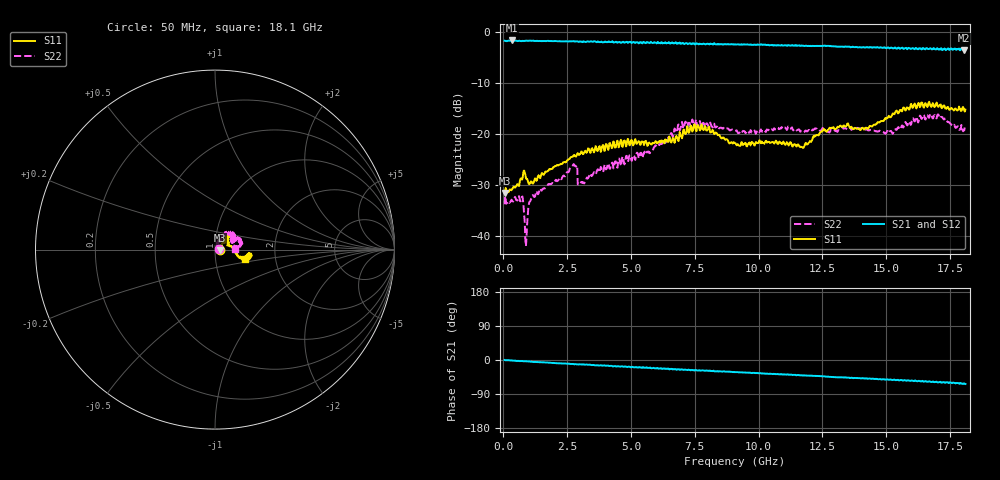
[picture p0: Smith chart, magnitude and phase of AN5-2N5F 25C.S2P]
! Network Analyzer HP8720D.06.14 Serial No. US36140669
! 12 Jan 2005  10:38:57
! Frequency  S11  S21  S12  S22
# HZ  S  DB R 50
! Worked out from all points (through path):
!   801 points, 50 MHz to 18.1 GHz, reference 50 ohm
!   highest |S21| = -1.60 dB at 343.3 MHz (marker M1); lowest = -3.5 dB at 18.03 GHz (marker M2)
!   group delay of S21, straight-line fit = 9.32 ps
!   lowest |S11| = -31.6 dB at 50 MHz (marker M3), VSWR 1.05, Z = 52.7 - j0.304 ohm
!   |S11| at or under -10 dB: start of sweep to end of sweep
!   |S22| runs from -42.0 to -16.0 dB; largest |S21 - S12| = 0.027
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5e7  -31.58 -6.3  -1.66 0.2  -1.68 -0.3  -33.79 4.1
3.433125e8  -30.75 12.3  -1.60 -1.5  -1.64 -1.7  -33.07 5.1
6.8175e8  -28.71 21.9  -1.72 -2.8  -1.70 -3.2  -33.19 10.7
8.848125e8  -28.68 10.7  -1.65 -3.3  -1.66 -3.7  -42.03 17.8
1.110438e9  -29.38 22.4  -1.69 -4.5  -1.61 -4.9  -32.62 53.3
2.689812e9  -24.50 39.6  -1.75 -10.4  -1.75 -10.7  -26.47 68.7
2.802625e9  -24.24 37.2  -1.84 -11.1  -1.80 -11.4  -26.29 67.3
3.005688e9  -23.93 44.7  -1.81 -11.7  -1.82 -12.0  -29.90 61.1
3.073375e9  -23.44 42.5  -1.85 -12.0  -1.80 -12.3  -29.43 64.3
4.810688e9  -22.43 39.7  -1.92 -17.4  -1.97 -18.1  -24.32 63.7
6.074188e9  -21.71 38.9  -2.04 -23.0  -2.02 -22.8  -22.39 61.3
7.202312e9  -18.45 47.2  -2.19 -26.6  -2.13 -26.2  -18.76 46.0
7.969438e9  -19.31 46.0  -2.25 -27.9  -2.26 -28.8  -17.87 34.2
9.075e9  -21.73 39.2  -2.38 -31.9  -2.31 -32.2  -19.35 25.7
1.169225e10  -22.51 19.4  -2.60 -40.5  -2.57 -40.9  -19.48 28.5
1.209838e10  -21.15 12.2  -2.66 -41.6  -2.63 -42.0  -19.22 32.7
1.284294e10  -18.87 -2.2  -2.70 -44.8  -2.67 -45.2  -19.14 31.1
1.421925e10  -18.75 -7.6  -2.93 -48.5  -2.88 -48.9  -19.13 27.9
1.509919e10  -16.41 -16.4  -3.07 -52.4  -2.93 -52.1  -19.77 28.1
1.667856e10  -13.66 -9.2  -3.29 -56.5  -3.09 -57.4  -16.80 17.7
1.803231e10  -14.98 -19.7  -3.54 -62.2  -3.56 -63.6  -19.31 10.3
1.81e10  -15.19 -17.0  -3.41 -63.3  -3.40 -63.8  -18.84 2.5
